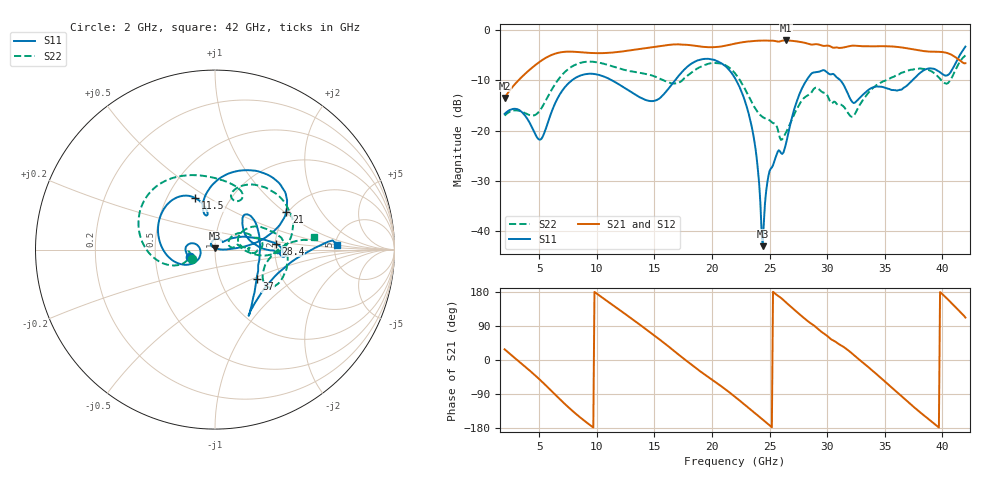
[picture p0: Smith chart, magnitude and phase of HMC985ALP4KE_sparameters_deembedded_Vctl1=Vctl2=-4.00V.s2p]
!s2p File: Measurements: S11, S21, S12, S22
# GHz S dB R 50.0
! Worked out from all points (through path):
!   401 points, 2 GHz to 42 GHz, reference 50 ohm
!   highest |S21| = -2.13 dB at 26.4 GHz (marker M1); lowest = -13.5 dB at 2 GHz (marker M2)
!   lowest |S11| = -42.9 dB at 24.4 GHz (marker M3), VSWR 1.01, Z = 50.1 + j0.706 ohm
!   |S11| at or under -10 dB: start of sweep to 7.866 GHz; 22.1 GHz to 28.21 GHz (6.118 GHz wide, 24.3 % of centre); 31.13 GHz to 37.41 GHz (6.275 GHz wide, 18.3 % of centre)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
!   |S22| runs from -21.9 to -5.1 dB; largest |S21 - S12| = 0.00065
!   S11 on the Smith chart (normalised r, x): 2 GHz: 0.75, -0.06; 11.5 GHz: 0.69, +0.44; 21 GHz: 1.95, +1.04; 28.4 GHz: 2.01, +0.15; 37 GHz: 1.49, -0.53; 42 GHz: 5.19, +0.54
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2  -16.69 -163.2  -13.52 28.2  -13.52 28.2  -17.03 -157.3
5.1  -21.79 -170.6  -6.28 -53.1  -6.28 -53.1  -15.89 -160.0
6.3  -15.03 -151.5  -4.82 -88.6  -4.82 -88.6  -11.08 -162.5
8.7  -8.99 149.7  -4.48 -154.9  -4.48 -154.9  -6.50 150.7
11.5  -10.27 110.8  -4.50 142.5  -4.50 142.5  -7.36 104.5
13.6  -13.22 101.7  -3.87 96.3  -3.88 96.3  -8.50 75.3
15.4  -13.70 106.7  -3.27 55.3  -3.27 55.3  -9.62 62.3
17.9  -7.25 79.2  -3.01 -4.9  -3.01 -4.9  -9.06 71.8
21  -6.94 28.1  -3.24 -73.5  -3.24 -73.5  -6.85 17.0
22  -9.59 16.5  -2.76 -97.1  -2.76 -97.1  -8.64 -0.2
23.5  -19.77 3.3  -2.26 -134.5  -2.26 -134.4  -14.56 -4.4
24.4  -42.92 80.0  -2.15 -157.2  -2.15 -157.1  -17.33 8.7
25  -28.04 125.6  -2.18 -172.5  -2.18 -172.5  -17.94 12.3
26.4  -22.81 41.4  -2.13 152.7  -2.13 152.7  -20.48 33.9
28.4  -9.37 5.7  -2.81 100.6  -2.81 100.6  -12.92 17.3
28.7  -8.58 0.7  -2.94 94.4  -2.95 94.4  -12.20 15.5
32.4  -14.48 30.9  -3.17 10.9  -3.16 10.8  -16.76 27.0
33.9  -11.50 47.5  -3.29 -27.2  -3.29 -27.2  -11.70 29.9
35.4  -11.76 17.0  -3.29 -67.3  -3.29 -67.3  -9.72 18.4
37  -10.92 -35.5  -3.71 -110.4  -3.71 -110.4  -8.11 3.7
39.8  -8.45 -55.4  -4.39 179.3  -4.39 179.3  -9.71 -33.8
42  -3.35 2.4  -6.64 111.9  -6.64 111.8  -5.09 7.4
